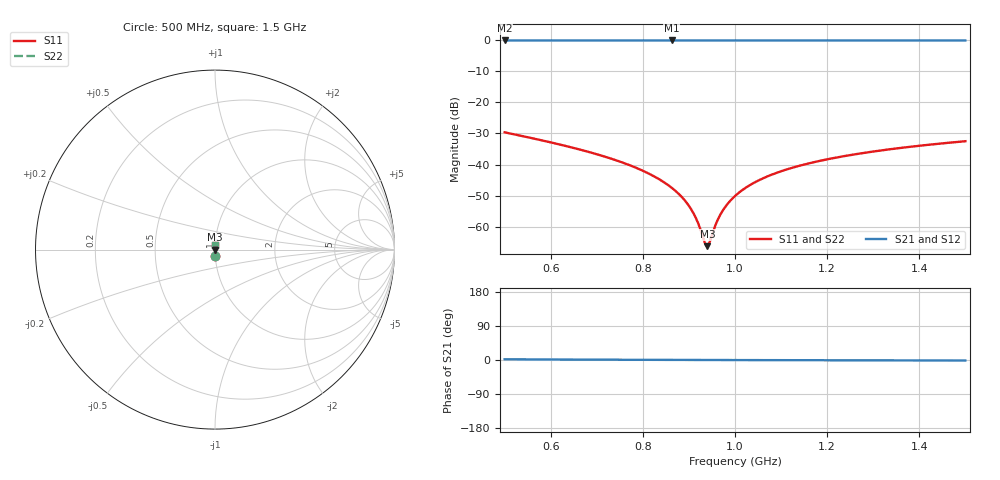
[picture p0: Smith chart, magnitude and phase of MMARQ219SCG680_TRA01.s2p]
! MMARQ219SCG680_TRA01  S-PARAMETER MODEL  ( General Type )
! Model Generated by TAIYO YUDEN Corporation (http://www.ty-top.com)
! Version 1.0
! TAIYO YUDEN Control No. 180601
! Copyright(c) 2018 TAIYO YUDEN CO.,LTD. All Rights Reserved.
! Product Description (link to TY-COMPAS)
! https://ds.yuden.co.jp/TYCOMPAS/or/detail?pn=MMARQ219SCG680JTRA01&u=M
! Products Name : Multilayer Ceramic Capacitors
! Characteristics :
!  Capacitance : 68 pF , Rated Voltage : 250V , TCC : CG / C0G
!  Case Size : 2.0 x 1.25 / 0.079 x 0.049 [mm/inch] , Thickness : 0.85 / 0.033 [mm/inch]
!  (Conditions: Temperature = 25 degC , DC Bias Current/Voltage = 0A / 0V)
! External Node Assignments :
!  1  o---| |---o  2
! GND o---------o GND
! Frequency Range : 500MHz  -  1500MHz  [ 401 STEP ]
# MHz S RI R 50
! Freq[MHz].  S11 Real  S11 Imag  S21 Real  S21 Imag  S12 Real  S12 Imag  S22 Real  S22 Imag
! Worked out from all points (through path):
!   401 points, 500 MHz to 1.5 GHz, reference 50 ohm
!   highest |S21| = 0.00 dB at 862.5 MHz (marker M1); lowest = 0.0 dB at 500 MHz (marker M2)
!   lowest |S11| = -66.3 dB at 940 MHz (marker M3), VSWR 1.00, Z = 50 + j0.00279 ohm
!   |S11| at or under -10 dB: start of sweep to end of sweep
!   |S22| runs from -66.3 to -29.6 dB; largest |S21 - S12| = 0
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500  0.00148 -0.033  0.9985 0.033  0.9985 0.033  0.00148 -0.033
667.5  0.00071 -0.0171  0.9993 0.0171  0.9993 0.0171  0.00071 -0.0171
765  0.000542 -0.0101  0.9995 0.0101  0.9995 0.0101  0.000542 -0.0101
835  0.000489 -0.00579  0.9995 0.00579  0.9995 0.00579  0.000489 -0.00579
862.5  0.00048 -0.00419  0.9995 0.00419  0.9995 0.00419  0.00048 -0.00419
887.5  0.000476 -0.00279  0.9995 0.00279  0.9995 0.00279  0.000476 -0.00279
905  0.000476 -0.00183  0.9995 0.00183  0.9995 0.00183  0.000476 -0.00183
917.5  0.000477 -0.00116  0.9995 0.00116  0.9995 0.00116  0.000477 -0.00116
935  0.00048 -0.000233  0.9995 0.000233  0.9995 0.000233  0.00048 -0.000233
940  0.000481 2.78e-05  0.9995 -2.78e-05  0.9995 -2.78e-05  0.000481 2.78e-05
945  0.000483 0.000288  0.9995 -0.000288  0.9995 -0.000288  0.000483 0.000288
960  0.000488 0.00106  0.9995 -0.00106  0.9995 -0.00106  0.000488 0.00106
970  0.000492 0.00157  0.9995 -0.00157  0.9995 -0.00157  0.000492 0.00157
982.5  0.000497 0.00219  0.9995 -0.00219  0.9995 -0.00219  0.000497 0.00219
1000  0.000507 0.00306  0.9995 -0.00306  0.9995 -0.00306  0.000507 0.00306
1027.5  0.000524 0.00439  0.9995 -0.00439  0.9995 -0.00439  0.000524 0.00439
1065  0.000553 0.00616  0.9994 -0.00616  0.9994 -0.00616  0.000553 0.00616
1110  0.000595 0.0082  0.9994 -0.0082  0.9994 -0.0082  0.000595 0.0082
1167.5  0.000659 0.0107  0.9993 -0.0107  0.9993 -0.0107  0.000659 0.0107
1242.5  0.000758 0.0139  0.9992 -0.0139  0.9992 -0.0139  0.000758 0.0139
1335  0.000902 0.0175  0.9991 -0.0175  0.9991 -0.0175  0.000902 0.0175
1500  0.00121 0.0237  0.9988 -0.0237  0.9988 -0.0237  0.00121 0.0237
